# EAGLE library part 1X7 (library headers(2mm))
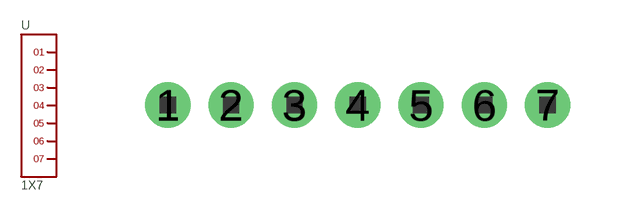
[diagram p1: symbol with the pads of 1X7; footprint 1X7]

Designator prefix -

## 1X7  [1X7]
1  1
2  2
3  3
4  4
5  5
6  6
7  7

## Footprint 1X7 (pad centres in mm)
drill 0.8 pad 1.422: 1 -6,0; 2 -4,0; 3 -2,0; 4 0,0; 5 2,0; 6 4,0; 7 6,0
